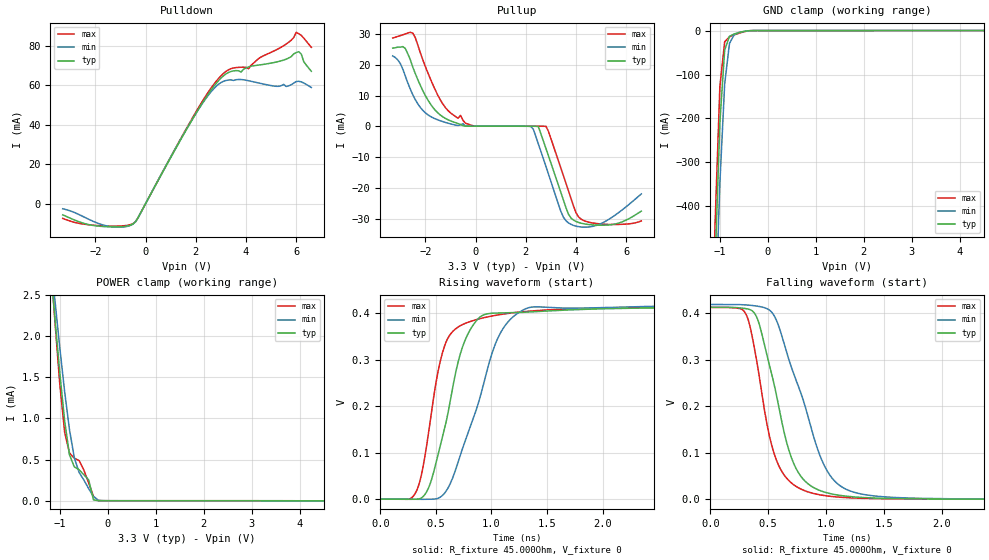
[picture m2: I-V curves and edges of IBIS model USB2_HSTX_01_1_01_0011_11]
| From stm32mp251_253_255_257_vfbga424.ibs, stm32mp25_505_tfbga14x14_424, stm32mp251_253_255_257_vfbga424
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[Model] USB2_HSTX_01_1_01_0011_11
Model_type   Output
Polarity   Non-Inverting
Enable   Active-High
C_comp   8.036pF   7.631pF   8.569pF
Vmeas = 200.000mV
Vref = 200.000mV
Rref = 45Ohms
Cref = 0pF
[Model Spec]
Vmeas   200.000mV   200.000mV   200.000mV
Vref   200.000mV   200.000mV   200.000mV
| This model is not intended for timing simulations.
| Warnings about Cref, Vref & Rref can be ignored
[Temperature Range]   25.000   125.000   -40.000
[Voltage Range]   3.300V   3.070V   3.630V
[GND Clamp Reference]   0.00V   0.00V   0.00V
[Pulldown Reference]   0.00V   0.00V   0.00V
[POWER Clamp Reference]   3.300V   3.070V   3.630V
[Pullup Reference]   3.300V   3.070V   3.630V
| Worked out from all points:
|   slope of the pulldown table from 0 to 0.495 V, typ, clamps not added: 42.6 ohm
|   GND clamp passes 1 mA (typ) near -0.43 V on its own axis
|   POWER clamp passes 1 mA (typ) near -0.91 V on its own axis
|   rising waveform, R_fixture 45.000Ohm, V_fixture 0: 20-80 % time 238ps typ, 332ps min, 184ps max; typ from 0 V to 0.413 V
|   falling waveform, R_fixture 45.000Ohm, V_fixture 0: 20-80 % time 242ps typ, 327ps min, 196ps max; typ from 0.413 V to 0 V
[GND Clamp]
-3.3V     -11.02A    -10.62A    -11.32A
-1.2V     -931.6mA   -1.049A    -855.7mA
-1.1V     -533.1mA   -671.7mA   -440.2mA
-1V       -209.4mA   -347mA     -127.3mA
-900mV    -44.44mA   -121.7mA   -25.6mA
-800mV    -13.15mA   -29.48mA   -14.15mA
-700mV    -7.743mA   -9.125mA   -9.769mA
-500mV    -2.127mA   -1.981mA   -2.894mA
-300mV    -19.53uA   -62.22uA   -13.67uA
6.6V      10.37uA    26.59uA    21.05uA
[Power Clamp]
-3.3V     3.206A     2.175A     4.855A
-1.2V     2.88mA     3.008mA    2.969mA
-1.1V     2.195mA    2.419mA    2.156mA
-1V       1.545mA    1.852mA    1.406mA
-900mV    966.9uA    1.324mA    831.4uA
-800mV    558.2uA    864.6uA    580.3uA
-700mV    412uA      525.9uA    517uA
-600mV    376.6uA    345uA      488.5uA
-400mV    254.2uA    146.6uA    216.8uA
-300mV    11.21uA    52.87uA    53.51uA
-100mV    94.86nA    985nA      361.1nA
6.6V      -2.431uA   -5.18uA    -3.436uA
[Pulldown]
-3.3V     -5.671mA   -2.581mA   -7.449mA
-1.6V     -11.64mA   -11.09mA   -11.31mA
-500mV    -10.25mA   -10.32mA   -10.1mA
1.9V      43.42mA    43.46mA    44.13mA
2.9V      62.15mA    60.37mA    63.26mA
3.4V      66.87mA    62.63mA    68.29mA
4.1V      69.19mA    62.19mA    68.26mA
4.5V      70.11mA    61.06mA    73.4mA
5.6V      73.12mA    59.29mA    80.76mA
6V        76.46mA    61.79mA    86.69mA
6.1V      76.88mA    61.92mA    85.99mA
6.6V      66.99mA    58.79mA    79.1mA
[Pullup]
-3.3V     25.41mA    22.87mA    28.67mA
-2.8V     25.31mA    16.38mA    30mA
-2.5V     19.21mA    10.28mA    30.28mA
-1.2V     2.603mA    1.31mA     6.11mA
-100mV    93.8uA     82.61uA    220.4uA
2.2V      68.65uA    -28.24uA   104.8uA
2.5V      -41.33uA   -5.658mA   83.46uA
2.9V      -9.472mA   -15.37mA   -1.562mA
3.5V      -23.92mA   -29.44mA   -16.02mA
3.8V      -29.68mA   -31.75mA   -23.35mA
4.4V      -31.68mA   -32.65mA   -30.79mA
6.6V      -27.44mA   -21.87mA   -30.63mA
[Ramp]
R_load=45.000Ohm
dV/dt_r   624.175mV/1.100ns  592.506mV/1.145ns  677.766mV/1.005ns
dV/dt_f   626.381mV/265.000ps  595.438mV/350.000ps  679.594mV/225.000ps
[Rising waveform]
R_fixture=45.000Ohm
V_fixture=0
0s        452.3nV    3.134uV    468nV
330ps     -200.2uV   -412.7uV   19.76mV
440ps     27.56mV    -306.8uV   152mV
510ps     86.29mV    1.143mV    262.8mV
580ps     153.7mV    13.3mV     331.1mV
750ps     334.5mV    116mV      377mV
970ps     399.4mV    285.5mV    392.7mV
1.13ns    401mV      376.1mV    399.3mV
1.38ns    403.5mV    413.9mV    405.6mV
9.9ns     413.1mV    419.2mV    412.8mV
[Falling waveform]
R_fixture=45.000Ohm
V_fixture=0
0s        412.6mV    418.6mV    412.3mV
310ps     409.6mV    417.6mV    396.7mV
410ps     385.7mV    414.9mV    283.8mV
540ps     258.8mV    398.9mV    107.4mV
650ps     130.9mV    323.5mV    48.1mV
720ps     76.95mV    269.7mV    31.26mV
960ps     17.63mV    85.68mV    9.061mV
1.17ns    6.839mV    21.89mV    3.692mV
1.66ns    1.372mV    3.243mV    934.1uV
9.9ns     13.77uV    30.91uV    4.011uV
